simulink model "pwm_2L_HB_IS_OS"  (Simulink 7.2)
settings: Solver=ode3  SolverMode=SingleTasking  StartTime=0.0  StopTime=0.1  FixedStep=10e-6  MaxStep=1e-4  RelTol=1e-3
PreLoadFcn:
  | INIT_PWM_2L
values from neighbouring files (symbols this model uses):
  VDC = 600    [INIT_PWM_2L.m]    (also in INIT_PWM_3L.m = 1200; INIT_PWM_Con.m = 1200; INIT_B6_2L_3Ph_IGBT_OS.m; INIT_B6_3L_3Ph_IGBT_OS.m = 1000)

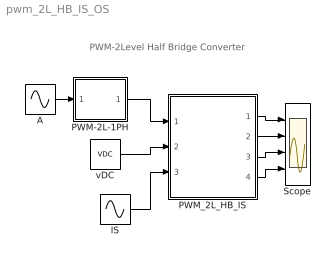
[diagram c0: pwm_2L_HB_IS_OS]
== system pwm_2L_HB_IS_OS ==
  note: PWM-2Level Half Bridge Converter
  A : Sin  Amplitude=0.5  Frequency=2*pi*50  Phase=[0]  SampleTime=0
  IS : Sin  Amplitude=400  Frequency=2*pi*50  Phase=[0]  SampleTime=0
  PWM-2L-1PH : Subsystem  mask(PWM-2L-1PH){FT=900, PHT=0, DT=1e-6}
      mask prompts: FT "Triangular Frequency"; PHT "Trian. Phase Angle (Degree)"; DT "Dead Time"
      mask help: Pulse Width Modulation for 1 Leg of 2-Level Converter
  PWM_2L_HB_IS : Subsystem
  Scope : Scope  NumInputPorts=4
  vDC : Constant  Value=VDC  OutDataType=sfix(16)  OutScaling=2^0
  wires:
  A/1 -> PWM-2L-1PH/1(In1)
  PWM_2L_HB_IS/1(vA) -> Scope/1
  vDC/1 -> PWM_2L_HB_IS/2(vDC)
  PWM-2L-1PH/1(Out1) -> PWM_2L_HB_IS/1(Sw)
  IS/1 -> PWM_2L_HB_IS/3(IS)
  PWM_2L_HB_IS/2(iA) -> Scope/2
  PWM_2L_HB_IS/3(iT1,iD1,vT1) -> Scope/3
  PWM_2L_HB_IS/4(iDC) -> Scope/4

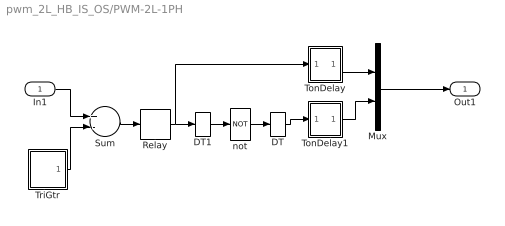
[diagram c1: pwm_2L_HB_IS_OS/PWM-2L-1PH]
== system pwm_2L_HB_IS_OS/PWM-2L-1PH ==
  In1 : Inport  OutDataType=sfix(16)  OutScaling=2^0
  DT : DataTypeConversion
  DT1 : DataTypeConversion
  Mux : Mux  Inputs=2
  Relay : Relay  OutDataType=sfix(16)  OutScaling=2^0
  Sum : Sum  Inputs=+-  OutDataType=sfix(16)  OutScaling=2^0
  TonDelay : Subsystem  mask(TonDelay){DT=DT}
      mask prompts: DT "Dead Time"
      mask help: Turn on dead time to protect against short circuit of the converter leg
  TonDelay1 : Subsystem  mask(TonDelay){DT=DT}
      mask prompts: DT "Dead Time"
      mask help: Turn on dead time to protect against short circuit of the converter leg
  TriGtr : Subsystem  mask(TriGtr){T=1/FT, Td=PHT/FT/360}
      mask prompts: T "Period Time"; Td "Time Delay"
      mask help: Triangular Wave Generator with variable time delay
  not : Logic  Operator=NOT  Inputs=1
  Out1 : Outport  InitialOutput=0
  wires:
  DT1/1 -> not/1
  DT/1 -> TonDelay1/1(s1)
  In1/1 -> Sum/1
  TriGtr/1(O) -> Sum/2
  Sum/1 -> Relay/1
  not/1 -> DT/1
  TonDelay1/1(s1d) -> Mux/2
  Relay/1 -> DT1/1, TonDelay/1(s1)
  TonDelay/1(s1d) -> Mux/1
  Mux/1 -> Out1/1

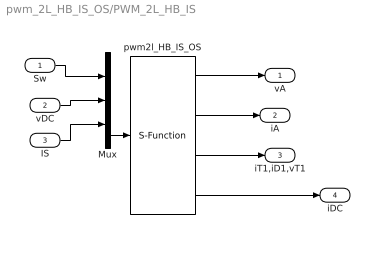
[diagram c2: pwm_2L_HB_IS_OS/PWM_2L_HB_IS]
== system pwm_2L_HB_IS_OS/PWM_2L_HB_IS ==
  Sw : Inport  OutDataType=sfix(16)  OutScaling=2^0
  vDC : Inport  Port=2  OutDataType=sfix(16)  OutScaling=2^0
  IS : Inport  Port=3  OutDataType=sfix(16)  OutScaling=2^0
  Mux : Mux  Inputs="[2  1  1]"
  pwm2l_HB_IS_OS : S-Function  FunctionName=s_pwm_2L_HB_IS_OS  Parameters=0  EnableBusSupport=off
  vA : Outport  OutDataType=sfix(16)  OutScaling=2^0
  iA : Outport  Port=2  OutDataType=sfix(16)  OutScaling=2^0
  iT1,iD1,vT1 : Outport  Port=3  OutDataType=sfix(16)  OutScaling=2^0
  iDC : Outport  Port=4  OutDataType=sfix(16)  OutScaling=2^0
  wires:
  pwm2l_HB_IS_OS/4 -> iDC/1
  pwm2l_HB_IS_OS/3 -> iT1,iD1,vT1/1
  pwm2l_HB_IS_OS/2 -> iA/1
  pwm2l_HB_IS_OS/1 -> vA/1
  IS/1 -> Mux/3
  Mux/1 -> pwm2l_HB_IS_OS/1
  vDC/1 -> Mux/2
  Sw/1 -> Mux/1

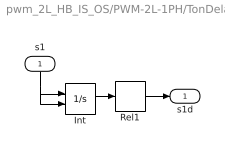
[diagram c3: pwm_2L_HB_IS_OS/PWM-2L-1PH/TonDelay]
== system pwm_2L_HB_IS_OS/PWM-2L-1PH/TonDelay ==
  s1 : Inport  Orientation=down  OutDataType=sfix(16)  OutScaling=2^0
  Int : Integrator  ExternalReset=falling
  Rel1 : Relay  OnSwitchValue=DT  OutDataType=sfix(16)  OutScaling=2^0
  s1d : Outport  InitialOutput=0
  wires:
  Int/1 -> Rel1/1
  s1/1 -> Int/2, Int/1
  Rel1/1 -> s1d/1

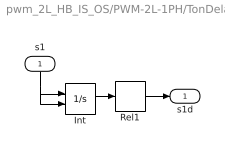
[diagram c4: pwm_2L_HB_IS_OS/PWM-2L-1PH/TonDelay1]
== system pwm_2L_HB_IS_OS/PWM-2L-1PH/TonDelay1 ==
  s1 : Inport  Orientation=down  OutDataType=sfix(16)  OutScaling=2^0
  Int : Integrator  ExternalReset=falling
  Rel1 : Relay  OnSwitchValue=DT  OutDataType=sfix(16)  OutScaling=2^0
  s1d : Outport  InitialOutput=0
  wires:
  Int/1 -> Rel1/1
  s1/1 -> Int/2, Int/1
  Rel1/1 -> s1d/1

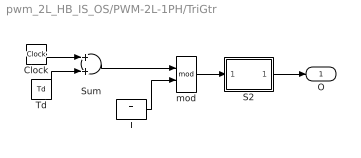
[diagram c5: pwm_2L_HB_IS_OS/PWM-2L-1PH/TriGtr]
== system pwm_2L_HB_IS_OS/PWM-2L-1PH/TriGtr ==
  Clock : Clock
  S2 : Subsystem
  Sum : Sum  OutDataType=sfix(16)  OutScaling=2^0
  T : Constant  Value=T  OutDataType=sfix(16)  OutScaling=2^0
  Td : Constant  Value=Td  OutDataType=sfix(16)  OutScaling=2^0
  mod : Math  Operator=mod
  O : Outport  InitialOutput=0
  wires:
  mod/1 -> S2/1(I1)
  S2/1(O1) -> O/1
  Clock/1 -> Sum/1
  T/1 -> mod/2
  Sum/1 -> mod/1
  Td/1 -> Sum/2

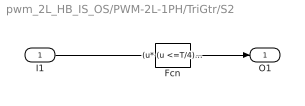
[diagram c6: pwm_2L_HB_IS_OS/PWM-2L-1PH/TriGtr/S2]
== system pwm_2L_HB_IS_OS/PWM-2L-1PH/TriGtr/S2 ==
  I1 : Inport
  Fcn : Fcn  Expr="(u* (u <=T/4) * 4/T)   +  (  (u > T/4) && ( u <=3*T/4) )* ( 1 - (u-T/4) *4/T )   +  ( (u > 3*T/4)&& (u<=T)) * ( ((u -3*T/4)* 4/T )-1 )"
  O1 : Outport
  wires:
  Fcn/1 -> O1/1
  I1/1 -> Fcn/1
